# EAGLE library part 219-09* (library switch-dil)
Surface Mount DIP Switch Series 219 SMT CTS Electronic Components Sourc: www.ctscorp.com
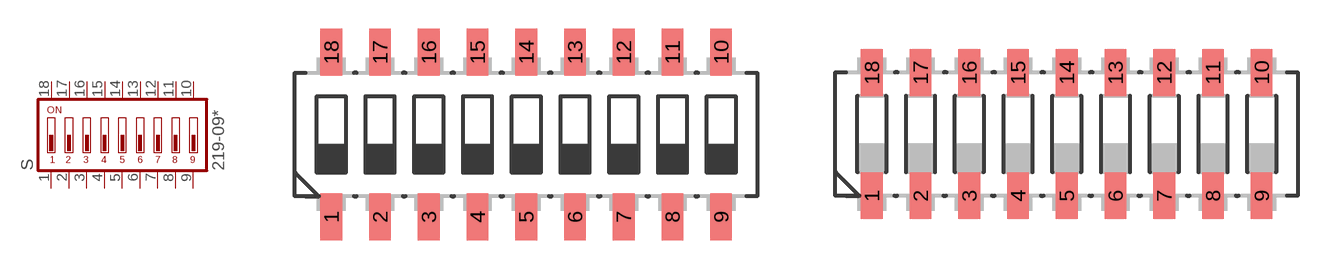
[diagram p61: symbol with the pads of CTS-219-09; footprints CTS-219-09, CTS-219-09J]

Designator prefix S

## 219-09 (OC_FARNELL: unknown; OC_NEWARK: unknown)  [CTS-219-09]
1  1  pas
2  2  pas
3  3  pas
4  4  pas
5  5  pas
6  6  pas
7  7  pas
8  8  pas
9  9  pas
10  10  pas
11  11  pas
12  12  pas
13  13  pas
14  14  pas
15  15  pas
16  16  pas
17  17  pas
18  18  pas

## 219-09J (OC_FARNELL: unknown; OC_NEWARK: unknown)  [CTS-219-09J]
Pads as for CTS-219-09

## Footprint CTS-219-09 (pad centres in mm)
Surface Mount DIP Switch Series 219 SMT CTS Electronic Components Sourc: www.ctscorp.com
smd 1.13 x 2.44: 1 -10.16,-4.3; 2 -7.62,-4.3; 3 -5.08,-4.3; 4 -2.54,-4.3; 5 0,-4.3; 6 2.54,-4.3; 7 5.08,-4.3; 8 7.62,-4.3; 9 10.16,-4.3; 10 10.16,4.3; 11 7.62,4.3; 12 5.08,4.3; 13 2.54,4.3; 14 0,4.3; 15 -2.54,4.3; 16 -5.08,4.3; 17 -7.62,4.3; 18 -10.16,4.3

## Footprint CTS-219-09J (pad centres in mm)
Surface Mount DIP Switch Series 219 SMT "J" Bend CTS Electronic Components Sourc: www.ctscorp.com
smd 1.13 x 2.44: 1 -10.16,-3.215; 2 -7.62,-3.215; 3 -5.08,-3.215; 4 -2.54,-3.215; 5 0,-3.215; 6 2.54,-3.215; 7 5.08,-3.215; 8 7.62,-3.215; 9 10.16,-3.215; 10 10.16,3.215; 11 7.62,3.215; 12 5.08,3.215; 13 2.54,3.215; 14 0,3.215; 15 -2.54,3.215; 16 -5.08,3.215; 17 -7.62,3.215; 18 -10.16,3.215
